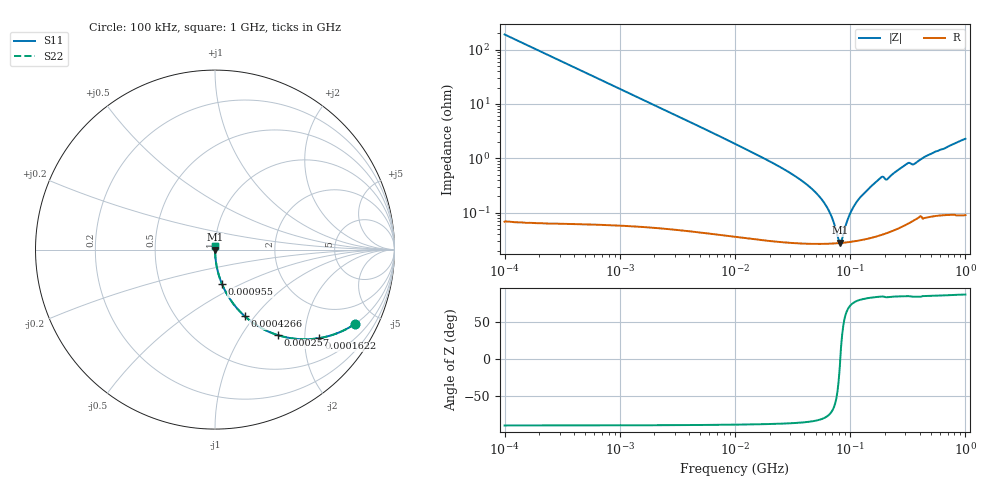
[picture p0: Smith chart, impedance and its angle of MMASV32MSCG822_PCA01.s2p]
! MMASV32MSCG822_PCA01  S-PARAMETER MODEL  ( Standard Model )
! Model Generated by TAIYO YUDEN Corporation (https://www.yuden.co.jp/en/)
! Version 1.0
! TAIYO YUDEN Control No. 250312
! Copyright(c) 2025 TAIYO YUDEN CO.,LTD. All Rights Reserved.
! Product Description (link to TY-COMPAS)
! https://ds.yuden.co.jp/TYCOMPAS/or/detail?pn=MMASV32MSCG822JPCA01&u=M
! Products Name : Multilayer Ceramic Capacitors
! Characteristics :
!  Capacitance : 8200 [pF] , Rated Voltage : 1000 [V] , TCC : CG / C0G
!  Case Size : 3.2 x 2.5 / 0.126 x 0.098 [mm/inch] , Thickness : 2.5 / 0.098 [mm/inch]
!  (Conditions: Temperature = 25 [degC] , DC Bias Voltage = 0 [V])
! External Node Assignments :
!  1  o---| |---o  2
! GND o---------o GND
! Frequency Range : 0.1MHz  -  1000MHz  [ 401 STEP ]
# MHZ S RI R 50
! Freq[MHz].  S11 Real  S11 Imag  S21 Real  S21 Imag  S12 Real  S12 Imag  S22 Real  S22 Imag
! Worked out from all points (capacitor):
!   401 points, 100 kHz to 1 GHz, reference 50 ohm
!   read as one part in series: C = 8.41 nF near 104.7 kHz
!   lowest |Z| = 28 mohm at 81.28 MHz (marker M1)
!   series resonance near 82.01 MHz, so ESL is about 450 pH
!   S11 on the Smith chart (normalised r, x): 100 kHz: 1.00, -3.79; 162.2 kHz: 1.00, -2.34; 257 kHz: 1.00, -1.47; 426.6 kHz: 1.00, -0.89; 955 kHz: 1.00, -0.40; 1 GHz: 1.00, +0.05
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0.1  0.7821 -0.4127  0.2179 0.4127  0.2179 0.4127  0.7821 -0.4127
0.162181  0.5768 -0.4938  0.4232 0.4938  0.4232 0.4938  0.5768 -0.4938
0.25704  0.3519 -0.4771  0.6481 0.4771  0.6481 0.4771  0.3519 -0.4771
0.42658  0.1649 -0.3704  0.8351 0.3704  0.8351 0.3704  0.1649 -0.3704
0.467735  0.1411 -0.3474  0.8589 0.3474  0.8589 0.3474  0.1411 -0.3474
0.954993  0.0384 -0.1906  0.9616 0.1906  0.9616 0.1906  0.0384 -0.1906
2.187762  0.00792 -0.0857  0.9921 0.0857  0.9921 0.0857  0.00792 -0.0857
10  0.000699 -0.0185  0.9993 0.0185  0.9993 0.0185  0.000699 -0.0185
26.91535  0.000322 -0.00619  0.9997 0.00619  0.9997 0.00619  0.000322 -0.00619
46.77351  0.000274 -0.00269  0.9997 0.00269  0.9997 0.00269  0.000274 -0.00269
63.09573  0.000269 -0.00121  0.9997 0.00121  0.9997 0.00121  0.000269 -0.00121
69.1831  0.00027 -0.000784  0.9997 0.000784  0.9997 0.000784  0.00027 -0.000784
77.62471  0.000274 -0.000257  0.9997 0.000257  0.9997 0.000257  0.000274 -0.000257
81.28305  0.000276 -4.85e-05  0.9997 4.85e-05  0.9997 4.85e-05  0.000276 -4.85e-05
85.1138  0.000278 0.00018  0.9997 -0.00018  0.9997 -0.00018  0.000278 0.00018
100  0.00029 0.000926  0.9997 -0.000926  0.9997 -0.000926  0.00029 0.000926
117.4898  0.000308 0.0017  0.9997 -0.0017  0.9997 -0.0017  0.000308 0.0017
181.9701  0.0004 0.00428  0.9996 -0.00428  0.9996 -0.00428  0.0004 0.00428
218.7762  0.000457 0.00448  0.9995 -0.00448  0.9995 -0.00448  0.000457 0.00448
309.0295  0.000667 0.00784  0.9993 -0.00784  0.9993 -0.00784  0.000667 0.00784
363.0781  0.000795 0.0079  0.9992 -0.0079  0.9992 -0.0079  0.000795 0.0079
1000  0.00142 0.0228  0.9986 -0.0228  0.9986 -0.0228  0.00142 0.0228
